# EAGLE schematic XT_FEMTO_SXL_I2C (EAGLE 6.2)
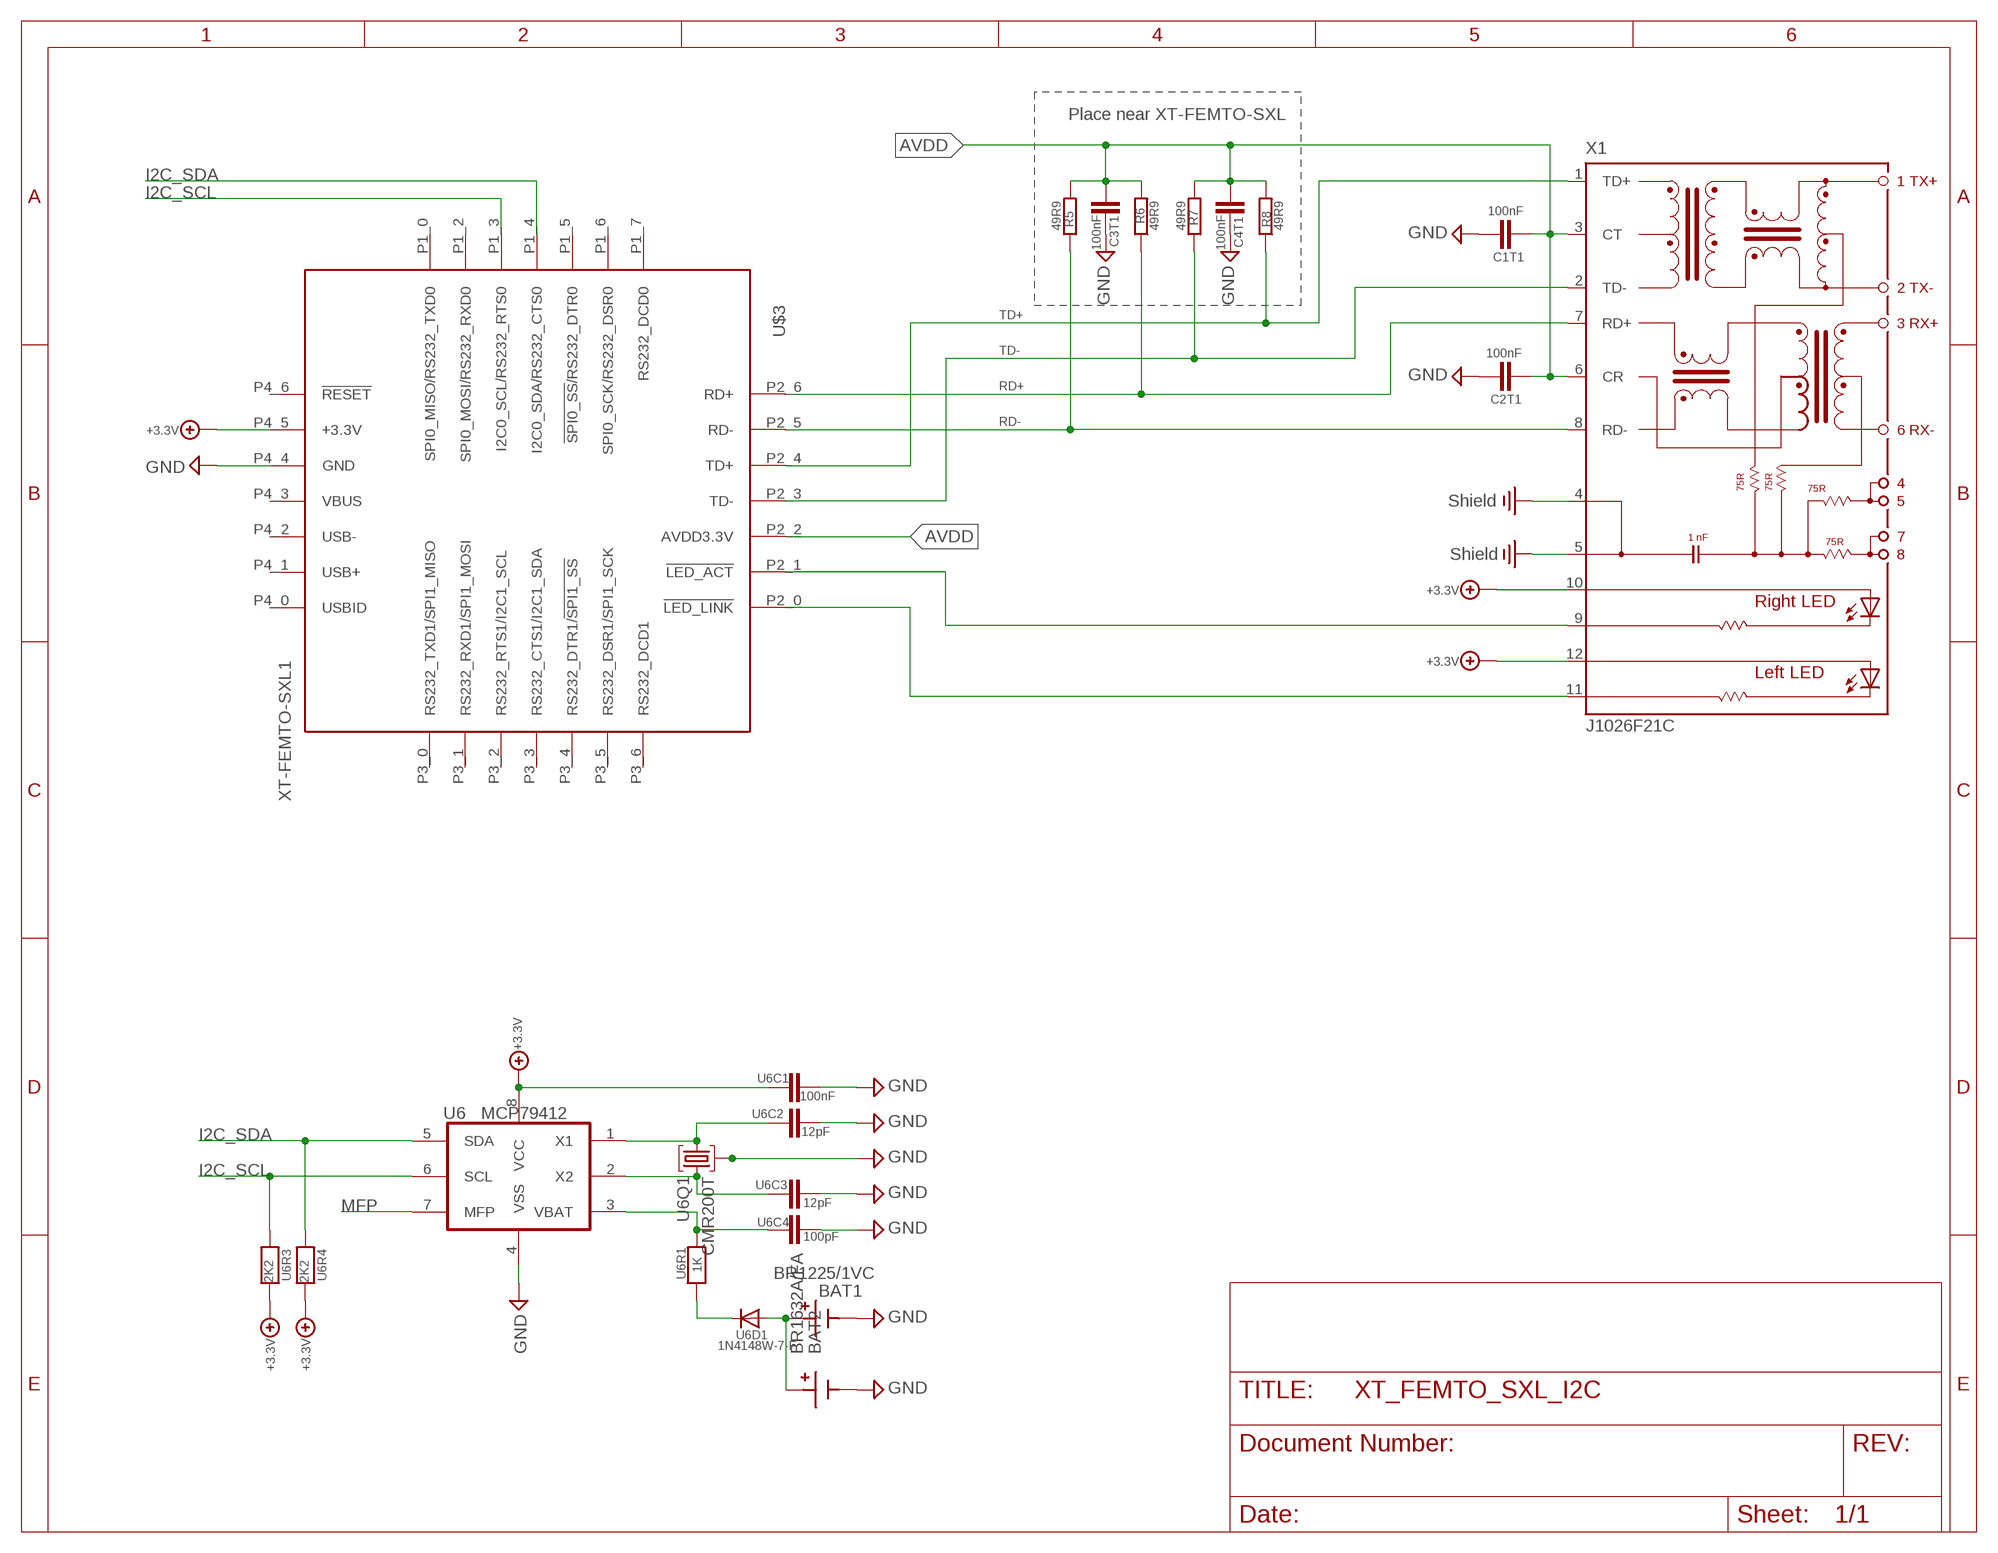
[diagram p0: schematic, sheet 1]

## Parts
BAT1  BR1225/1VC  [BR1225VC]
BAT2  BR1632A/FA  [BR1632A/FA]
C1T1  100nF  CHIP-C-VTS0402  [R0402_VTS]
C2T1  100nF  CHIP-C-VTS0402  [R0402_VTS]
C3T1  100nF  CHIP-C-VTS0402  [R0402_VTS]
C4T1  100nF  CHIP-C-VTS0402  [R0402_VTS]
R5  49R9  R-EU_R0603  [R0603]
R6  49R9  R-EU_R0603  [R0603]
R7  49R9  R-EU_R0603  [R0603]
R8  49R9  R-EU_R0603  [R0603]
U6  MCP79412  [SO-8]
U6C1  100nF  CHIP-C-VTS0402  [R0402_VTS]
U6C2  12pF  CHIP-C-VTS0402  [R0402_VTS]
U6C3  12pF  CHIP-C-VTS0402  [R0402_VTS]
U6C4  100pF  CHIP-C-VTS0402  [R0402_VTS]
U6D1  1N4148W-7-F  DIODE-SOD123  [SOD123]
U6Q1  CMR200T  [CMR200T]
U6R1  1K  CHIP-R-VTS04020402_VTS  [R0402_VTS@2]
U6R3  2K2  CHIP-R-VTS04020402_VTS  [R0402_VTS@2]
U6R4  2K2  CHIP-R-VTS04020402_VTS  [R0402_VTS@2]
U$3  XT-FEMTO-SXL1  [XT-FEMTO-SXL-PIN]
X1  J1026F21C  [J1]

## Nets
+3.3V: U6.8(VCC) U6C1.1 U6R3.2 U6R4.2 U$3.P4_5(+3.3V) X1.10(A-R) X1.12(A-L)
AVDD: C1T1.1 C2T1.2 C3T1.1 C4T1.2 R5.2 R6.2 R7.2 R8.2 U$3.P2_2(AVDD3.3V) X1.3(CT) X1.6(CR)
GND: BAT1.2 BAT2.P- C1T1.2 C2T1.1 C3T1.2 C4T1.1 U6.4(VSS) U6C1.2 U6C2.1 U6C3.1 U6C4.2 U6Q1.EXP U$3.P4_4(GND)
I2C_SCL: U6.6(SCL) U6R3.1 U$3.P1_3(I2C0_SCL/RS232_RTS0)
I2C_SDA: U6.5(SDA) U6R4.1 U$3.P1_4(I2C0_SDA/RS232_CTS0)
MFP: U6.7(MFP)
N$3: U$3.P2_1(!LED_ACT) X1.9(C-R)
N$5: U$3.P2_0(!LED_LINK) X1.11(C-L)
N$30: U6.2(X2) U6C3.2 U6Q1.2
N$34: U6.1(X1) U6C2.2 U6Q1.1
N$36: U6.3(VBAT) U6C4.1 U6R1.2
N$45: U6D1.C U6R1.1
N$46: BAT1.1 BAT2.P+ U6D1.A
PE: X1.4 X1.5 ; supply symbol labelled Shield
RD+: R6.1 U$3.P2_6(RD+) X1.7(RD+)
RD-: R5.1 U$3.P2_5(RD-) X1.8(RD-)
TD+: R8.1 U$3.P2_4(TD+) X1.1(TD+)
TD-: R7.1 U$3.P2_3(TD-) X1.2(TD-)
Unconnected: U$3.P1_0(SPI0_MISO/RS232_TXD0) U$3.P1_2(SPI0_MOSI/RS232_RXD0) U$3.P1_5(!SPI0_SS!/RS232_DTR0) U$3.P1_6(SPI0_SCK/RS232_DSR0) U$3.P1_7(RS232_DCD0) U$3.P3_0(RS232_TXD1/SPI1_MISO) U$3.P3_1(RS232_RXD1/SPI1_MOSI) U$3.P3_2(RS232_RTS1/I2C1_SCL) U$3.P3_3(RS232_CTS1/I2C1_SDA) U$3.P3_4(RS232_DTR1/!SPI1_SS!) U$3.P3_5(RS232_DSR1/SPI1_SCK) U$3.P3_6(RS232_DCD1) U$3.P4_0(USBID) U$3.P4_1(USB+) U$3.P4_2(USB-) U$3.P4_3(VBUS) U$3.P4_6(!RESET)

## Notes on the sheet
- Place near XT-FEMTO-SXL

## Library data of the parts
BAT1 = ak-nord:BR1225/1VC: Panasonic BR-1225/VCN Lithium Battery 3V 48mAh 12,5mm
BAT2 = ak-nord:BR1632A/FA: Panasonic BR1632A/FA Lithium Battery 3V 120mAh d=16mm
C1T1 C2T1 C3T1 C4T1 U6C1-U6C4 = mea-lib:CHIP-C-?: Chip capacitance
R5-R8 = rcl:R-EU_: RESISTOR, European symbol
U6 = ak-nord:MCP79412: I2C Real-Time Clock/Calendar with EEPROM, SRAM, Unique ID and Battery Switchover
U6D1 = diode:DIODE-: DIODE
U6Q1 = ak-nord:CMR200T
U6R1 U6R3 U6R4 = mea-lib:CHIP-R-?: Chip resistors
U$3 = ak-devices:XT-FEMTO-SXL: AK-NORD XT-FEMTO-SXL
X1 = con-pulse:J1026F: PULSEJACK (TM) 1x1 Tab-UP RJ45 10/100 Base-TX RJ45 1x1 Tab-UP with LEDs 8-pin (J1 series) and 6-pin (JP series) integrated magnetics connector, designed to support applications, such as ADSL modems, LAN-on-Motherboard, and Hub and Switches. Source: www.pulseeng.com .. PulseJack-J402.pdf; OC_FARNELL: unknown; OC_NEWARK: unknown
